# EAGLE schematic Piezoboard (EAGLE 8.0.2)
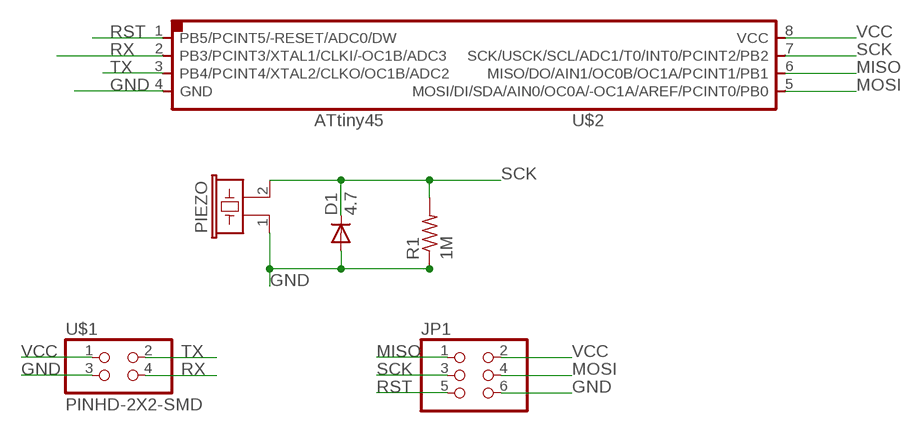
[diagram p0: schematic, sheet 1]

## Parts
D1  4.7  DIODESOD123  [SOD123]
JP1  PINHD-2X3-SMD  [2X03SMD]
PIEZO  EFBAA40D101  [EFBAA40D101]
R1  1M  RES-US1206FAB  [R1206FAB]
U$1  PINHD-2X2-SMD  [2X02SMD]
U$2  ATTINY45SI  [SOIC8]

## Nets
GND: D1.ANODE(A) JP1.6 PIEZO.1 R1.1 U$1.3 U$2.4(GND)
MISO: JP1.1 U$2.6(MISO/DO/AIN1/OC0B/OC1A/PCINT1/PB1)
MOSI: JP1.4 U$2.5(MOSI/DI/SDA/AIN0/OC0A/-OC1A/AREF/PCINT0/PB0)
RST: JP1.5 U$2.1(PB5/PCINT5/-RESET/ADC0/DW)
RX: U$1.4 U$2.2(PB3/PCINT3/XTAL1/CLKI/-OC1B/ADC3)
SCK: D1.CATHODE(C) JP1.3 PIEZO.2 R1.2 U$2.7(SCK/USCK/SCL/ADC1/T0/INT0/PCINT2/PB2)
TX: U$1.2 U$2.3(PB4/PCINT4/XTAL2/CLKO/OC1B/ADC2)
VCC: JP1.2 U$1.1 U$2.8(VCC)

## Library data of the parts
D1 = fab:DIODE: DIODE
JP1 = 01_FAB_Hello:PINHD-2X3-SMD: PIN HEADER
PIEZO = buzzer:EFB?: Piezoelectric Acoustic Transducer; OC_FARNELL: unknown; OC_NEWARK: unknown
R1 = fab:RES-US: Resistor (US Symbol)
U$1 = fab:PINHD-2X2-SMD
U$2 = 01_fab:ATTINY45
